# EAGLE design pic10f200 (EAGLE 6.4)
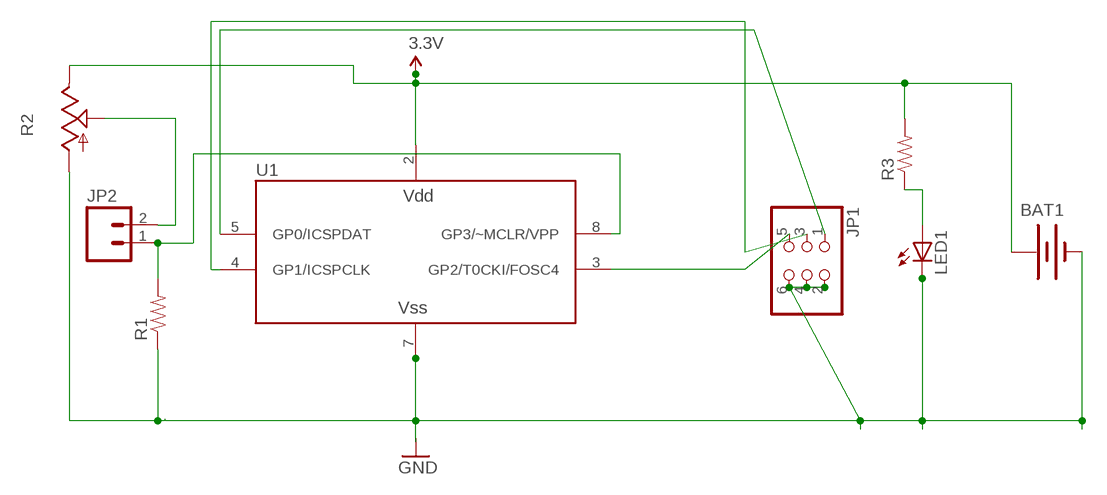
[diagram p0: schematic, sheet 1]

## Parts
BAT1  BATTERY20PTH  [BATTCOM_20MM_PTH]
JP1  PINHD-2X3  [2X03]
JP2  M02PTH  [1X02]
LED1  LED-3MM-NO_SILK  [LED3MM-NS]
R1  RESISTORKIT  [AXIAL-0.3-KIT]
R2  TRIM_US-B25U  [B25U]
R3  RESISTORKIT  [AXIAL-0.3-KIT]
U1  PIC10F200P  [DIP-8]

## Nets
3.3V: BAT1.1(+) R2.E R3.P$2 U1.2(VDD)
N$1: JP2.1 R1.P$2 U1.8(GP3/~MCLR/VPP)
N$2: JP1.1 U1.5(GP0/ICSPDAT)
N$3: LED1.A R3.P$1
N$4: JP1.5 U1.3(GP2/T0CKI/FOSC4)
N$5: JP1.3 U1.4(GP1/ICSPCLK)
N$6: JP2.2 R2.S
N$7: BAT1.2(-) JP1.2 JP1.4 JP1.6 LED1.K(C) R1.P$1 R2.A U1.7(VSS)

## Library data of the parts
BAT1 = SparkFun:BATTERY: Battery Holders
JP1 = SparkFun:PINHD-2X3: PIN HEADER
JP2 = SparkFun:M02: Header 2
LED1 = SparkFun:LED: LEDs
R1 R3 = SparkFun:RESISTOR: Resistor
R2 = pot:TRIM_US-: POTENTIOMETER
U1 = microchip_2:PIC10F20*: Microchip PIC10F200, 202, 204 and 206 6-pin 8-bit Flash microcontroller 256/512 words program memory, 16/24 bytes RAM 4 I/O, 1 8-bit timer, 1 comparator on PIC10F204 and PIC10F206

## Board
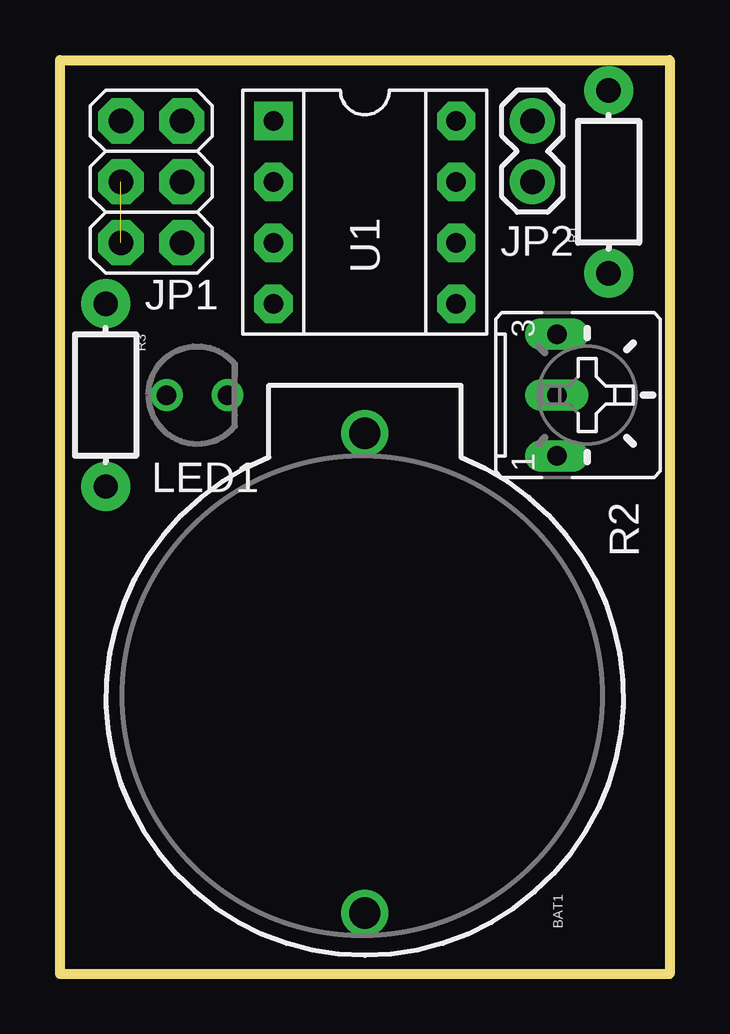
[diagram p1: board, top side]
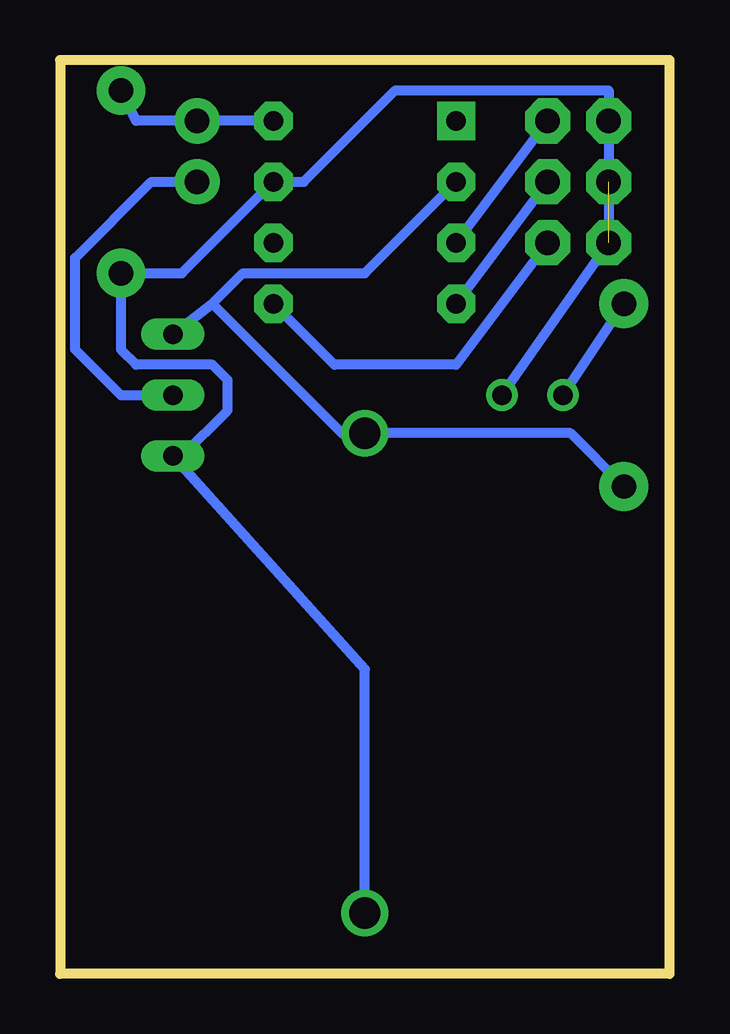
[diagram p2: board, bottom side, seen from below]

Size 25.4 x 38.1 mm. Coordinates in mm from the lower left corner, seen from the top.
Outline: 0,0 0,38.1 25.4,38.1 25.4,0 0,0
Copper layers (1*16): Top 0.035mm / dielectric 1.5mm / Bottom 0.035mm
Design rules "default": minimum track width 10mil, minimum drill 0.6mm, track to track 8mil, track to pad 8mil, pad to pad 8mil, via to via 8mil, smd to smd 8mil, copper to edge 40mil, drill to drill 8mil, minimum pad ring 10mil, minimum via ring 8mil, stop-mask expansion 4mil, vias tented up to drill 0mil, thermal gap 10mil

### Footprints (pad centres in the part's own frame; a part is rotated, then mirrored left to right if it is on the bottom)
BATTCOM_20MM_PTH = drill 1.3: 1 20,0; 2 0,0
2X03 = drill 1.016 pad 1.88 octagon: 1 -2.54,-1.27; 2 -2.54,1.27; 3 0,-1.27; 4 0,1.27; 5 2.54,-1.27; 6 2.54,1.27
1X02 = drill 1.016 pad 1.88: 1 0,0; 2 2.54,0
LED3MM-NS = drill 0.813: A -1.27,0; K 1.27,0
AXIAL-0.3-KIT = drill 1.016 pad 2.032: P$1 -3.81,0; P$2 3.81,0
B25U = drill 0.813 long: A 2.54,-0.889; E -2.54,-0.889; S 0,-0.889
DIP-8 = drill 0.813 pad 1.6 square: 1 -3.81,3.81 | drill 0.813 pad 1.6 octagon: 2 -3.81,1.27; 3 -3.81,-1.27; 4 -3.81,-3.81; 5 3.81,-3.81; 6 3.81,-1.27; 7 3.81,1.27; 8 3.81,3.81

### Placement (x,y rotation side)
BAT1  12.7,2.54 90 top
JP1  3.81,33.02 90 top
JP2  19.68,35.56 270 top
LED1  5.71,24.13 0 top
R1  22.86,33.02 90 top
R2  21.59,24.13 270 top
R3  1.9,24.13 270 top
U1  12.7,31.75 0 top

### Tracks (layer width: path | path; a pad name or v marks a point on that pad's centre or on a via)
3.3V
  Bottom 0.406: R3.P$2 4.12,22.54 BAT1.1 13.65,22.54 19.05,27.94 | R2.E 19.05,27.94 | 19.05,27.94 17.78,29.21 12.7,29.21 U1.2
N$1
  Bottom 0.406: U1.8 JP2.1 22.22,35.56 R1.P$2
N$2
  Bottom 0.406: JP1.1 8.89,25.4 13.97,25.4 U1.5
N$3
  Bottom 0.406: R3.P$1 LED1.A
N$4
  Bottom 0.406: U1.3 JP1.5
N$5
  Bottom 0.406: JP1.3 U1.4
N$6
  Bottom 0.406: 21.59,24.13 R2.S 22.86,24.13 24.76,26.04 24.76,29.84 21.59,33.02 JP2.2
N$7  (1 unrouted)
  Bottom 0.406: BAT1.2 12.7,12.7 R2.A 20.32,21.59 18.41,23.5 18.41,24.77 19.05,25.4 22.22,25.4 22.86,26.04 R1.P$1 20.32,29.21 U1.7 | LED1.K JP1.2 JP1.6 2.54,36.83 11.43,36.83 15.24,33.02 U1.7 | 17,32.75 U1.7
